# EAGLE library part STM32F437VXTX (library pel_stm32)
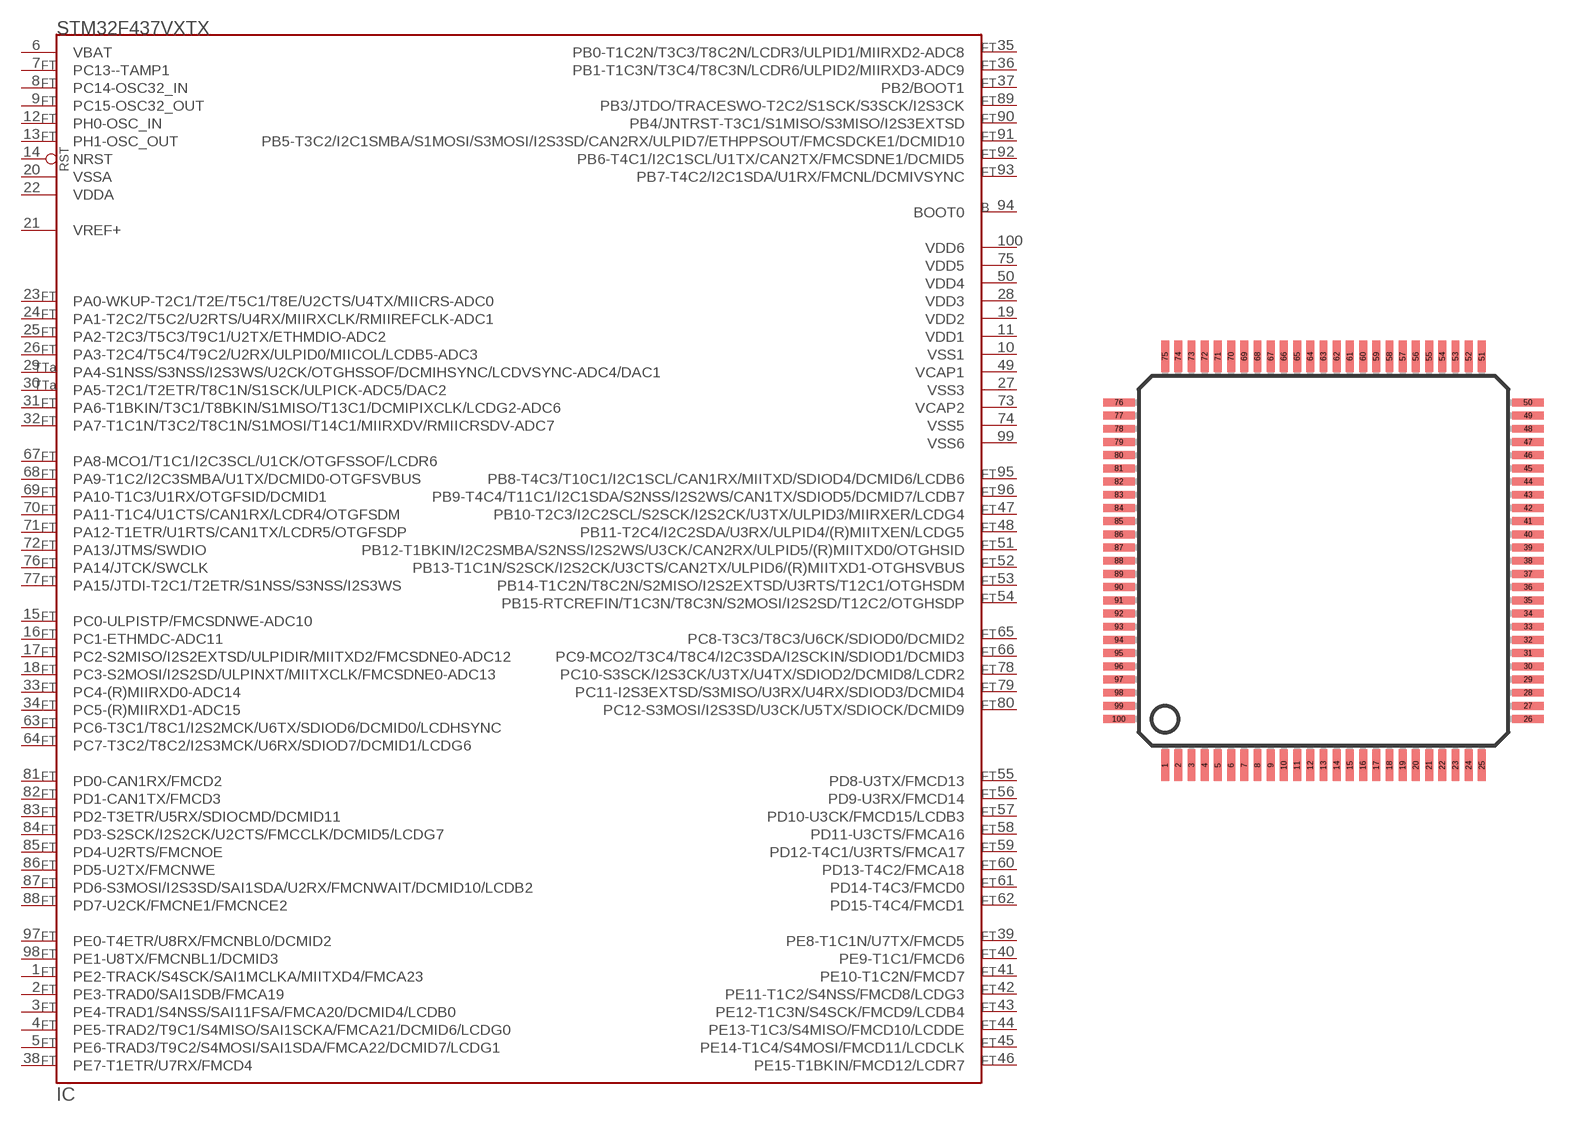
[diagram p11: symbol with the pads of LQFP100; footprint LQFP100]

Designator prefix IC

## STM32F437VXTX  [LQFP100]
1  PE2-TRACK/S4SCK/SAI1MCLKA/MIITXD4/FMCA23
2  PE3-TRAD0/SAI1SDB/FMCA19
3  PE4-TRAD1/S4NSS/SAI11FSA/FMCA20/DCMID4/LCDB0
4  PE5-TRAD2/T9C1/S4MISO/SAI1SCKA/FMCA21/DCMID6/LCDG0
5  PE6-TRAD3/T9C2/S4MOSI/SAI1SDA/FMCA22/DCMID7/LCDG1
6  VBAT  pwr
7  PC13--TAMP1
8  PC14-OSC32_IN
9  PC15-OSC32_OUT
10  VSS1  pwr
11  VDD1  pwr
12  PH0-OSC_IN  in
13  PH1-OSC_OUT
14  NRST
15  PC0-ULPISTP/FMCSDNWE-ADC10
16  PC1-ETHMDC-ADC11
17  PC2-S2MISO/I2S2EXTSD/ULPIDIR/MIITXD2/FMCSDNE0-ADC12
18  PC3-S2MOSI/I2S2SD/ULPINXT/MIITXCLK/FMCSDNE0-ADC13
19  VDD2  pwr
20  VSSA  pwr
21  VREF+
22  VDDA  pwr
23  PA0-WKUP-T2C1/T2E/T5C1/T8E/U2CTS/U4TX/MIICRS-ADC0
24  PA1-T2C2/T5C2/U2RTS/U4RX/MIIRXCLK/RMIIREFCLK-ADC1
25  PA2-T2C3/T5C3/T9C1/U2TX/ETHMDIO-ADC2
26  PA3-T2C4/T5C4/T9C2/U2RX/ULPID0/MIICOL/LCDB5-ADC3
27  VSS3  pwr
28  VDD3  pwr
29  PA4-S1NSS/S3NSS/I2S3WS/U2CK/OTGHSSOF/DCMIHSYNC/LCDVSYNC-ADC4/DAC1
30  PA5-T2C1/T2ETR/T8C1N/S1SCK/ULPICK-ADC5/DAC2
31  PA6-T1BKIN/T3C1/T8BKIN/S1MISO/T13C1/DCMIPIXCLK/LCDG2-ADC6
32  PA7-T1C1N/T3C2/T8C1N/S1MOSI/T14C1/MIIRXDV/RMIICRSDV-ADC7
33  PC4-(R)MIIRXD0-ADC14
34  PC5-(R)MIIRXD1-ADC15
35  PB0-T1C2N/T3C3/T8C2N/LCDR3/ULPID1/MIIRXD2-ADC8
36  PB1-T1C3N/T3C4/T8C3N/LCDR6/ULPID2/MIIRXD3-ADC9
37  PB2/BOOT1
38  PE7-T1ETR/U7RX/FMCD4
39  PE8-T1C1N/U7TX/FMCD5
40  PE9-T1C1/FMCD6
41  PE10-T1C2N/FMCD7
42  PE11-T1C2/S4NSS/FMCD8/LCDG3
43  PE12-T1C3N/S4SCK/FMCD9/LCDB4
44  PE13-T1C3/S4MISO/FMCD10/LCDDE
45  PE14-T1C4/S4MOSI/FMCD11/LCDCLK
46  PE15-T1BKIN/FMCD12/LCDR7
47  PB10-T2C3/I2C2SCL/S2SCK/I2S2CK/U3TX/ULPID3/MIIRXER/LCDG4
48  PB11-T2C4/I2C2SDA/U3RX/ULPID4/(R)MIITXEN/LCDG5
49  VCAP1  pwr
50  VDD4  pwr
51  PB12-T1BKIN/I2C2SMBA/S2NSS/I2S2WS/U3CK/CAN2RX/ULPID5/(R)MIITXD0/OTGHSID
52  PB13-T1C1N/S2SCK/I2S2CK/U3CTS/CAN2TX/ULPID6/(R)MIITXD1-OTGHSVBUS
53  PB14-T1C2N/T8C2N/S2MISO/I2S2EXTSD/U3RTS/T12C1/OTGHSDM
54  PB15-RTCREFIN/T1C3N/T8C3N/S2MOSI/I2S2SD/T12C2/OTGHSDP
55  PD8-U3TX/FMCD13
56  PD9-U3RX/FMCD14
57  PD10-U3CK/FMCD15/LCDB3
58  PD11-U3CTS/FMCA16
59  PD12-T4C1/U3RTS/FMCA17
60  PD13-T4C2/FMCA18
61  PD14-T4C3/FMCD0
62  PD15-T4C4/FMCD1
63  PC6-T3C1/T8C1/I2S2MCK/U6TX/SDIOD6/DCMID0/LCDHSYNC
64  PC7-T3C2/T8C2/I2S3MCK/U6RX/SDIOD7/DCMID1/LCDG6
65  PC8-T3C3/T8C3/U6CK/SDIOD0/DCMID2
66  PC9-MCO2/T3C4/T8C4/I2C3SDA/I2SCKIN/SDIOD1/DCMID3
67  PA8-MCO1/T1C1/I2C3SCL/U1CK/OTGFSSOF/LCDR6
68  PA9-T1C2/I2C3SMBA/U1TX/DCMID0-OTGFSVBUS
69  PA10-T1C3/U1RX/OTGFSID/DCMID1
70  PA11-T1C4/U1CTS/CAN1RX/LCDR4/OTGFSDM
71  PA12-T1ETR/U1RTS/CAN1TX/LCDR5/OTGFSDP
72  PA13/JTMS/SWDIO
73  VCAP2  pwr
74  VSS5  pwr
75  VDD5  pwr
76  PA14/JTCK/SWCLK
77  PA15/JTDI-T2C1/T2ETR/S1NSS/S3NSS/I2S3WS
78  PC10-S3SCK/I2S3CK/U3TX/U4TX/SDIOD2/DCMID8/LCDR2
79  PC11-I2S3EXTSD/S3MISO/U3RX/U4RX/SDIOD3/DCMID4
80  PC12-S3MOSI/I2S3SD/U3CK/U5TX/SDIOCK/DCMID9
81  PD0-CAN1RX/FMCD2
82  PD1-CAN1TX/FMCD3
83  PD2-T3ETR/U5RX/SDIOCMD/DCMID11
84  PD3-S2SCK/I2S2CK/U2CTS/FMCCLK/DCMID5/LCDG7
85  PD4-U2RTS/FMCNOE
86  PD5-U2TX/FMCNWE
87  PD6-S3MOSI/I2S3SD/SAI1SDA/U2RX/FMCNWAIT/DCMID10/LCDB2
88  PD7-U2CK/FMCNE1/FMCNCE2
89  PB3/JTDO/TRACESWO-T2C2/S1SCK/S3SCK/I2S3CK
90  PB4/JNTRST-T3C1/S1MISO/S3MISO/I2S3EXTSD
91  PB5-T3C2/I2C1SMBA/S1MOSI/S3MOSI/I2S3SD/CAN2RX/ULPID7/ETHPPSOUT/FMCSDCKE1/DCMID10
92  PB6-T4C1/I2C1SCL/U1TX/CAN2TX/FMCSDNE1/DCMID5
93  PB7-T4C2/I2C1SDA/U1RX/FMCNL/DCMIVSYNC
94  BOOT0  in
95  PB8-T4C3/T10C1/I2C1SCL/CAN1RX/MIITXD/SDIOD4/DCMID6/LCDB6
96  PB9-T4C4/T11C1/I2C1SDA/S2NSS/I2S2WS/CAN1TX/SDIOD5/DCMID7/LCDB7
97  PE0-T4ETR/U8RX/FMCNBL0/DCMID2
98  PE1-U8TX/FMCNBL1/DCMID3
99  VSS6  pwr
100  VDD6  pwr

## Footprint LQFP100 (pad centres in mm)
smd 0.3 x 1.2: 1 -6,-7.75; 2 -5.5,-7.75; 3 -5,-7.75; 4 -4.5,-7.75; 5 -4,-7.75; 6 -3.5,-7.75; 7 -3,-7.75; 8 -2.5,-7.75; 9 -2,-7.75; 10 -1.5,-7.75; 11 -1,-7.75; 12 -0.5,-7.75; 13 0,-7.75; 14 0.5,-7.75; 15 1,-7.75; 16 1.5,-7.75; 17 2,-7.75; 18 2.5,-7.75; 19 3,-7.75; 20 3.5,-7.75; 21 4,-7.75; 22 4.5,-7.75; 23 5,-7.75; 24 5.5,-7.75; 25 6,-7.75; 51 6,7.75; 52 5.5,7.75; 53 5,7.75; 54 4.5,7.75; 55 4,7.75; 56 3.5,7.75; 57 3,7.75; 58 2.5,7.75; 59 2,7.75; 60 1.5,7.75; 61 1,7.75; 62 0.5,7.75; 63 0,7.75; 64 -0.5,7.75; 65 -1,7.75; 66 -1.5,7.75; 67 -2,7.75; 68 -2.5,7.75; 69 -3,7.75; 70 -3.5,7.75; 71 -4,7.75; 72 -4.5,7.75; 73 -5,7.75; 74 -5.5,7.75; 75 -6,7.75
smd 1.2 x 0.3: 26 7.75,-6; 27 7.75,-5.5; 28 7.75,-5; 29 7.75,-4.5; 30 7.75,-4; 31 7.75,-3.5; 32 7.75,-3; 33 7.75,-2.5; 34 7.75,-2; 35 7.75,-1.5; 36 7.75,-1; 37 7.75,-0.5; 38 7.75,0; 39 7.75,0.5; 40 7.75,1; 41 7.75,1.5; 42 7.75,2; 43 7.75,2.5; 44 7.75,3; 45 7.75,3.5; 46 7.75,4; 47 7.75,4.5; 48 7.75,5; 49 7.75,5.5; 50 7.75,6; 76 -7.75,6; 77 -7.75,5.5; 78 -7.75,5; 79 -7.75,4.5; 80 -7.75,4; 81 -7.75,3.5; 82 -7.75,3; 83 -7.75,2.5; 84 -7.75,2; 85 -7.75,1.5; 86 -7.75,1; 87 -7.75,0.5; 88 -7.75,0; 89 -7.75,-0.5; 90 -7.75,-1; 91 -7.75,-1.5; 92 -7.75,-2; 93 -7.75,-2.5; 94 -7.75,-3; 95 -7.75,-3.5; 96 -7.75,-4; 97 -7.75,-4.5; 98 -7.75,-5; 99 -7.75,-5.5; 100 -7.75,-6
